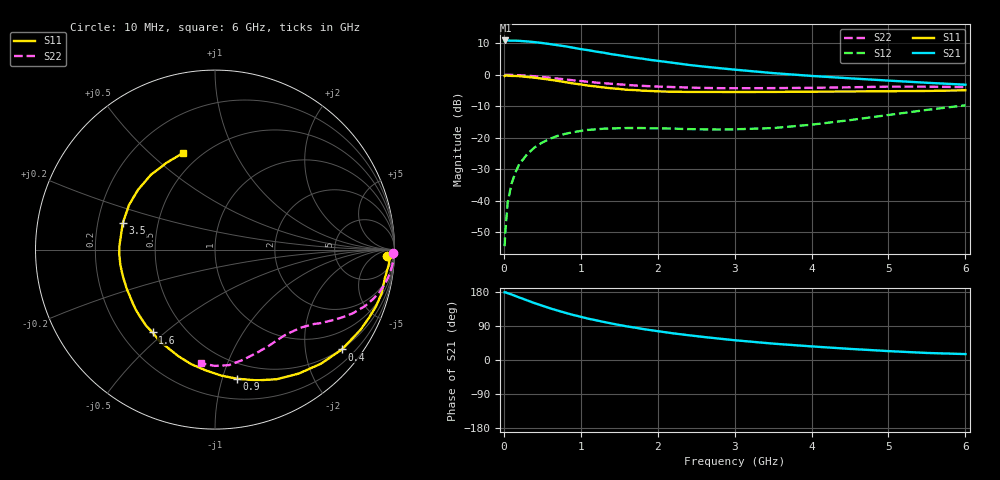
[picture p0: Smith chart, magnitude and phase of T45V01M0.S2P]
! Infineon Technologies  Discrete & RF Semiconductors
! BFR182T
! Si NPN RF Bipolar Junction Transistor in SC75
! VCE = 5 V  IC = 1 mA
! Common Emitter S-Parameters:  October  1999
# GHz  S  MA  R  50
!  f  S11  S21  S12  S22
! GHz  MAG  ANG  MAG  ANG  MAG  ANG  MAG  ANG
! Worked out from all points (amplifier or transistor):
!   36 points, 10 MHz to 6 GHz, reference 50 ohm
!   highest |S21| = 10.9 dB at 20 MHz (marker M1)
!   |S21| within 3 dB of that: start of sweep to 1.072 GHz
!   unconditionally stable (mu >= 1): 2.404 GHz to 4.579 GHz
!   at 250 MHz: K = 0.09, MSG = 18.8 dB, |S12| = -26.9 dB
!   at 1.4 GHz: K = 0.58, MSG = 11.8 dB, |S12| = -17.0 dB
!   at 6 GHz: K = 0.83, MSG = 3.3 dB, |S12| = -9.7 dB
!   S11 on the Smith chart (normalised r, x): 10 MHz: 27, -23; 400 MHz: 0.48, -2.81; 900 MHz: 0.36, -1.12; 1.6 GHz: 0.33, -0.45; 3.5 GHz: 0.31, +0.13; 6 GHz: 0.40, +0.64
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0.01  0.9576 -2.1  3.48 178.7  0.0019 82.2  0.9906 -1.1
0.02  0.9792 -0.8  3.51 178.8  0.0033 93.9  0.9999 -0.8
0.05  0.9714 -5.1  3.502 176.3  0.0094 89.1  0.9965 -1.9
0.1  0.9601 -9.3  3.477 172.9  0.0187 84.5  0.995 -3.8
0.15  0.9594 -14.8  3.481 168.9  0.0281 81.4  0.9895 -5.6
0.2  0.9516 -19.3  3.457 165.0  0.0381 79.2  0.9837 -7.5
0.3  0.9256 -28.9  3.386 157.6  0.0544 73.7  0.9685 -11.0
0.4  0.8997 -38.2  3.303 150.0  0.0703 67.9  0.9476 -14.4
0.5  0.8677 -47.1  3.195 143.2  0.0841 62.7  0.9234 -17.3
0.6  0.8337 -55.9  3.075 136.5  0.0966 58.4  0.8972 -20.2
0.8  0.7648 -72.3  2.833 124.5  0.1156 50.6  0.8446 -24.9
0.9  0.7296 -80.4  2.693 119.0  0.1226 47.1  0.8182 -26.9
1.1  0.6731 -94.9  2.457 108.9  0.1335 41.5  0.7732 -30.3
1.4  0.6096 -114.7  2.124 96.3  0.1406 35.1  0.7197 -34.6
1.6  0.578 -127.0  1.949 88.7  0.1429 32.5  0.6903 -36.9
1.8  0.5604 -138.1  1.804 82.0  0.1429 31.1  0.6669 -39.5
2.2  0.538 -155.8  1.549 70.4  0.1399 30.4  0.6388 -44.0
2.8  0.5339 -176.8  1.276 56.4  0.1352 34.7  0.6138 -51.9
3.5  0.5344 164.1  1.064 43.2  0.1426 45.4  0.6146 -61.1
4.5  0.5432 142.1  0.879 29.3  0.1908 58.2  0.6332 -75.5
5.5  0.5538 119.2  0.747 18.6  0.2772 60.4  0.6479 -90.1
6  0.5672 108.3  0.696 15.6  0.3277 57.9  0.6378 -97.0
